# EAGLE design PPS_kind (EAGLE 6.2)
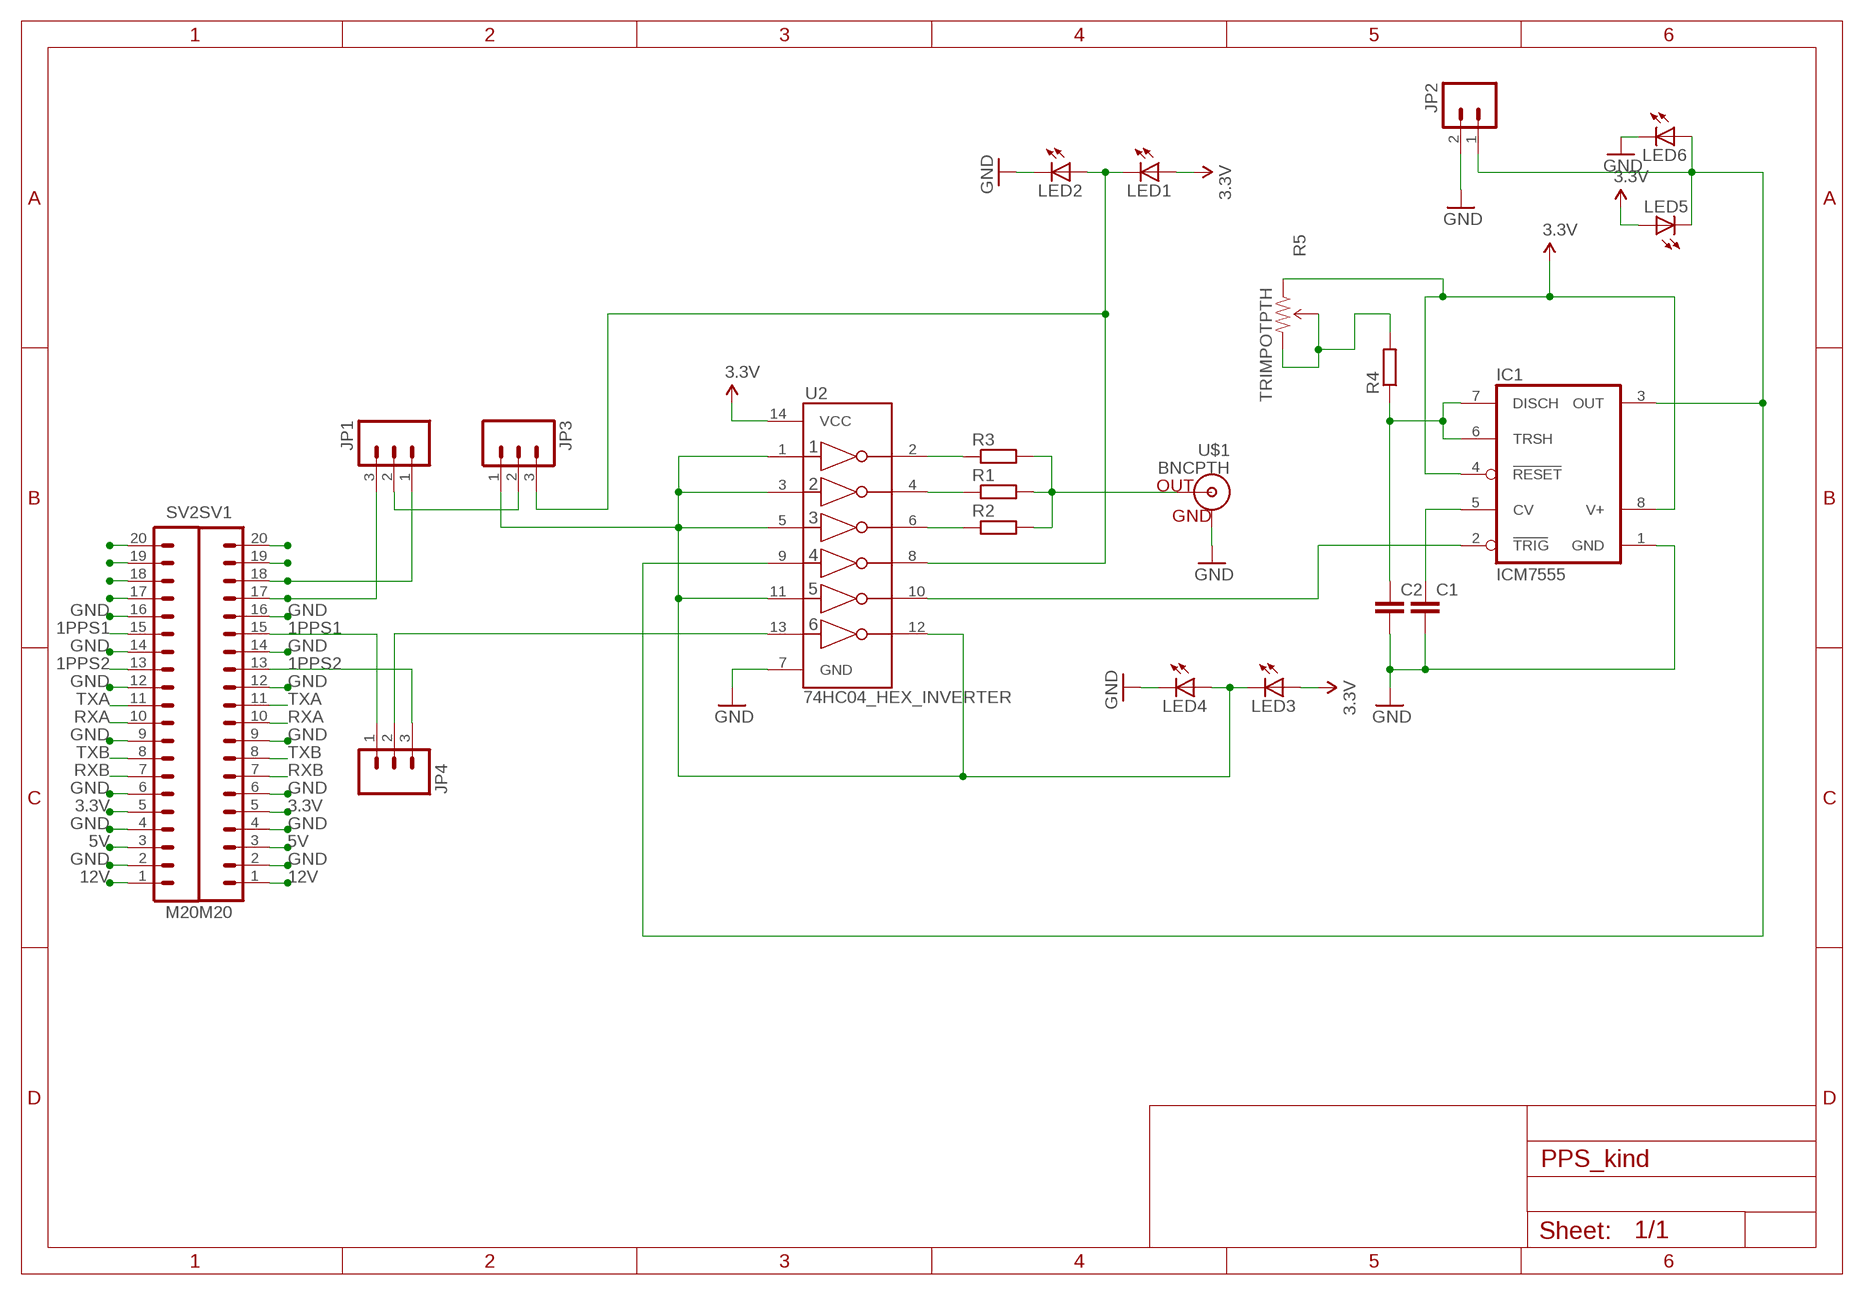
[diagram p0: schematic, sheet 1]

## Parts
C1  CAPPTH1  [CAP-PTH-5MM]
C2  CAPPTH1  [CAP-PTH-5MM]
IC1  ICM7555  [DIL08]
JP1  M03LONGPADS  [1X03_LONGPADS]
JP2  M02PTH3  [1X02_LONGPADS]
JP3  M03LONGPADS  [1X03_LONGPADS]
JP4  M03LONGPADS  [1X03_LONGPADS]
LED1  LED5MM  [LED5MM]
LED2  LED5MM  [LED5MM]
LED3  LED5MM  [LED5MM]
LED4  LED5MM  [LED5MM]
LED5  LED5MM  [LED5MM]
LED6  LED5MM  [LED5MM]
R1  R-EU_0207/10  [0207/10]
R2  R-EU_0207/10  [0207/10]
R3  R-EU_0207/10  [0207/10]
R4  R-EU_0204/2V  [0204V]
R5  TRIMPOTPTH  [TRIM_POT_PTH]
SV1  M20  [1X20]
SV2  M20  [1X20]
U2  74HC04_HEX_INVERTER  [DIL14]
U$1  BNCPTH  [BNC]

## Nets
1PPS1: JP4.1 SV1.15 SV2.15
1PPS2: JP4.3 SV1.13 SV2.13
3.3V: IC1.4(RESET) IC1.8(V+) LED1.A LED3.A LED5.A R5.1(CCW) SV1.5 SV2.5 U2.14(VCC)
5V: SV1.3 SV2.3
12V: SV1.1 SV2.1
GND: C1.2 C2.2 IC1.1(GND) JP2.2 LED2.K(C) LED4.K(C) LED6.K(C) SV1.2 SV1.4 SV1.6 SV1.9 SV1.12 SV1.14 SV1.16 SV2.2 SV2.4 SV2.6 SV2.9 SV2.12 SV2.14 SV2.16 U2.7(GND) U$1.GND
N$1: C1.1 IC1.5(CV)
N$2: JP4.2 U2.13(6A)
N$3: SV2.17
N$4: SV2.18
N$5: SV2.19
N$6: SV2.20
N$8: IC1.2(TRIG) U2.10(5Y)
N$9: JP3.1 LED3.K(C) LED4.A U2.1(1A) U2.3(2A) U2.5(3A) U2.11(5A) U2.12(6Y)
N$10: JP1.2 JP3.2
N$11: IC1.3(OUT) JP2.1 LED5.K(C) LED6.A U2.9(4A)
N$12: JP3.3 LED1.K(C) LED2.A U2.8(4Y)
N$13: R4.2 R5.2(WIPER) R5.3(CW)
N$15: R1.1 U2.4(2Y)
N$16: R2.1 U2.6(3Y)
N$17: JP1.3 SV1.17
N$18: JP1.1 SV1.18
N$19: SV1.19
N$20: SV1.20
N$21: R3.1 U2.2(1Y)
N$24: R1.2 R2.2 R3.2 U$1.S(OUT)
N$25: C2.1 IC1.6(TRSH) IC1.7(DISCH) R4.1
RXA: SV1.10 SV2.10
RXB: SV1.7 SV2.7
TXA: SV1.11 SV2.11
TXB: SV1.8 SV2.8

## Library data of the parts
C1 C2 = SparkFun:CAP: Capacitor
IC1 = maxim:ICM7555: TIMER; MF: MAXIM; MPN: ICM7555IPA+; OC_FARNELL: 9663762; OC_NEWARK: 68K4387
JP1 JP3 JP4 = SparkFun:M03: Header 3 Standard 3-pin 0.1" header. Use with straight break away headers (SKU : PRT-00116), right angle break away headers (PRT-00553), swiss pins (PRT-00743), machine pins (PRT-00117), and female headers (PRT-00115). Molex polarized connector foot print use with SKU : PRT-08232 with associated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
JP2 = SparkFun:M02: Header 2
LED1-LED6 = SparkFun:LED: LEDs
R1-R4 = rcl:R-EU_: RESISTOR, European symbol
R5 = SparkFun:TRIMPOT
SV1 SV2 = SparkFun:M20: This is just like the LOCK variant in that the holes are staggared by 5 mil, but except for the last two holes. They are not altered from the "standard" footprint layout. This is used for a special purpose on the layout of our Graphic LCD Backpack. Make sure you want to use this device before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
U2 = SparkFun:74HC04_HEX_INVERTER: 74HC04 Hex Inverter
U$1 = SparkFun:BNC: BNC Connector, Mouser Part# 5227161

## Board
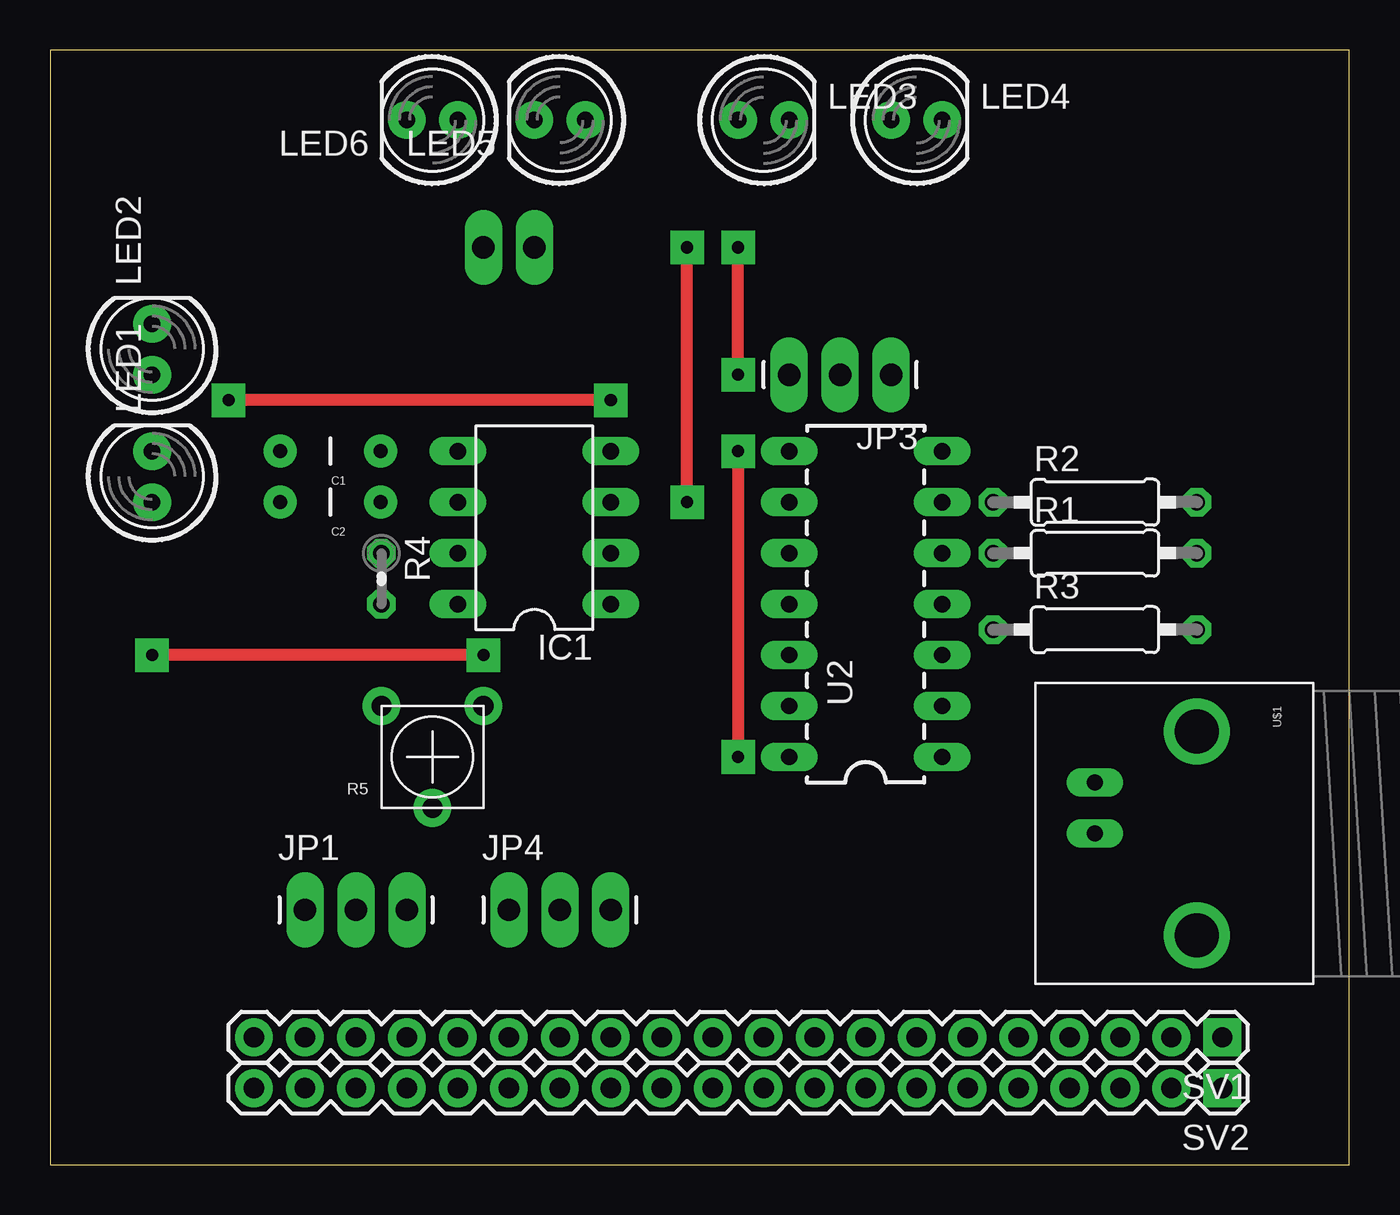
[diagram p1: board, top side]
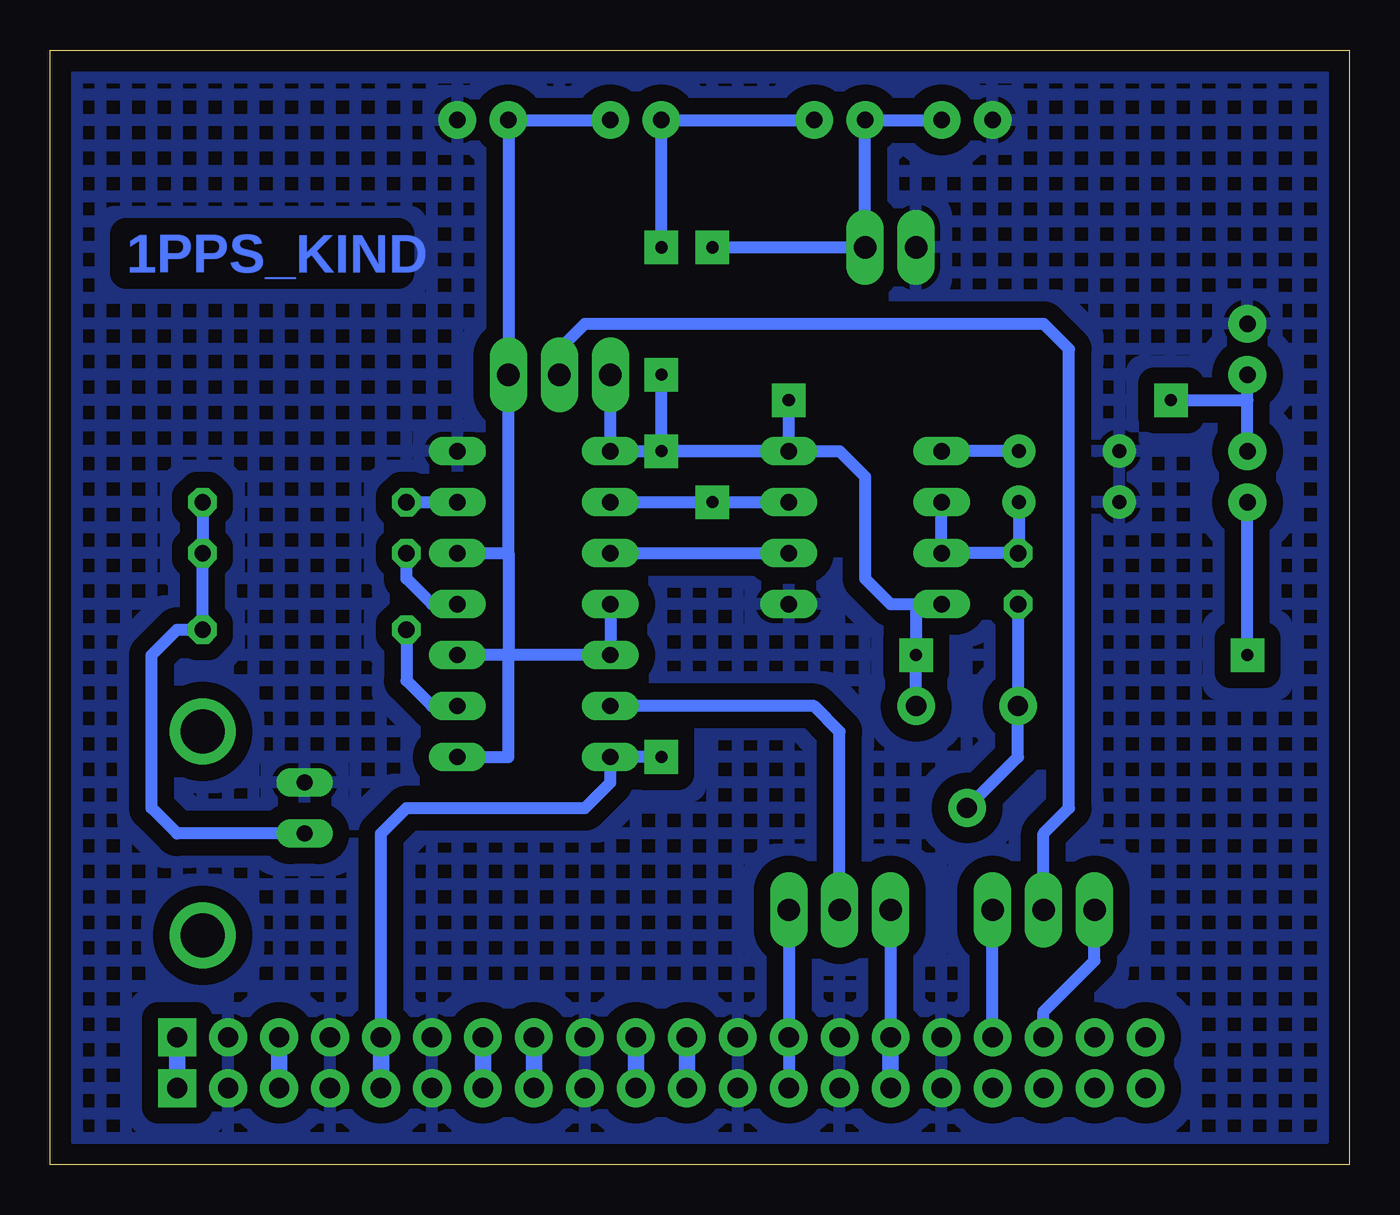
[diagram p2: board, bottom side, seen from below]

Size 64.75 x 55.55 mm. Coordinates in mm from the lower left corner, seen from the top.
Outline: 0,0 64.75,0 64.75,55.55 0,55.55 0,0
Copper layers (1*16): Top 0.035mm / dielectric 1.5mm / Bottom 0.035mm
Design rules: minimum track width 10mil, minimum drill 24mil, track to track 8mil, track to pad 8mil, pad to pad 8mil, via to via 8mil, smd to smd 8mil, copper to edge 40mil, drill to drill 8mil, minimum pad ring 12mil, minimum via ring 12mil, stop-mask expansion 4mil, vias tented up to drill 0mil, thermal gap 10mil

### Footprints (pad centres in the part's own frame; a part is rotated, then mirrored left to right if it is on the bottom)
CAP-PTH-5MM = drill 0.7 pad 1.651: 1 -2.5,0; 2 2.5,0
DIL08 = drill 0.813 long: 1 -3.81,-3.81; 2 -1.27,-3.81; 3 1.27,-3.81; 4 3.81,-3.81; 5 3.81,3.81; 6 1.27,3.81; 7 -1.27,3.81; 8 -3.81,3.81
1X03_LONGPADS = drill 1.118 pad 1.88 long: 1 0,0; 2 2.54,0; 3 5.08,0
1X02_LONGPADS = drill 1.118 pad 1.88 long: 1 0,0; 2 2.54,0
LED5MM = drill 0.813 pad 1.88: A -1.27,0; K 1.27,0
0207/10 = drill 0.813 octagon: 1 -5.08,0; 2 5.08,0
0204V = drill 0.813 octagon: 1 -1.27,0; 2 1.27,0
TRIM_POT_PTH = drill 1 pad 1.88: 1 -2.54,-2.54; 2 0,2.54; 3 2.54,-2.54
1X20 = drill 1.016 pad 1.88 square: 1 0,0 | drill 1.016 pad 1.88: 2 2.54,0; 3 5.08,0; 4 7.62,0; 5 10.16,0; 6 12.7,0; 7 15.24,0; 8 17.78,0; 9 20.32,0; 10 22.86,0; 11 25.4,0; 12 27.94,0; 13 30.48,0; 14 33.02,0; 15 35.56,0; 16 38.1,0; 17 40.64,0; 18 43.18,0; 19 45.72,0; 20 48.26,0
DIL14 = drill 0.813 long: 1 -8.89,-3.81; 2 -6.35,-3.81; 3 -3.81,-3.81; 4 -1.27,-3.81; 5 1.27,-3.81; 6 3.81,-3.81; 7 6.35,-3.81; 8 6.35,3.81; 9 3.81,3.81; 10 1.27,3.81; 11 -1.27,3.81; 12 -3.81,3.81; 13 -6.35,3.81; 14 -8.89,3.81
BNC = drill 2.2: 3 -5.08,5.08; 4 5.08,5.08 | drill 0.8 long: GND -2.54,0; S 0,0

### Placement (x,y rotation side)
C1  13.97,35.56 180 top
C2  13.97,33.02 180 top
IC1  24.13,31.75 90 top
JP1  12.7,12.7 0 top
JP2  24.13,45.72 180 top
JP3  41.91,39.37 180 top
JP4  22.86,12.7 0 top
LED1  5.08,34.29 90 top
LED2  5.08,40.64 90 top
LED3  35.56,52.07 0 top
LED4  43.18,52.07 0 top
LED5  25.4,52.07 180 top
LED6  19.05,52.07 180 top
R1  52.07,30.48 0 top
R2  52.07,33.02 0 top
R3  52.07,26.67 0 top
R4  16.51,29.21 270 top
R5  19.05,20.32 180 top
SV1  58.42,6.35 180 top
SV2  58.42,3.81 180 top
U2  40.64,29.21 90 top
U$1  52.07,16.51 270 top

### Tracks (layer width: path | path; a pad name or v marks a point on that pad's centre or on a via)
1PPS1
  Bottom 0.61: JP4.1 SV2.15
  Bottom 0.813: SV1.15 SV2.15
1PPS2
  Bottom 0.61: JP4.3 SV1.13 SV2.13
3.3V  (via drill 0.6, 0.6 pad 1.68)
  Top 0.61: v34.29,35.56 v34.29,20.32 | v21.59,25.4 v5.08,25.4 | v34.29,39.37 v34.29,45.72
  Bottom 0.61: v34.29,20.32 U2.14 36.83,19.05 38.1,17.78 46.99,17.78 48.26,16.51 SV1.5 | 21.59,27.94 22.86,27.94 24.13,29.21 24.13,34.29 25.4,35.56 IC1.4 v34.29,35.56 v34.29,39.37 | R5.1 v21.59,25.4 21.59,27.94 | LED5.A LED3.A v34.29,45.72 | IC1.8 21.59,27.94 | v5.08,25.4 LED1.A
  Bottom 0.813: SV1.5 SV2.5
5V
  Bottom 0.813: SV1.3 SV2.3
12V
  Bottom 0.813: SV1.1 SV2.1
GND
  pour Bottom (isolate 0.813, hatched): 1.27,1.27 1.27,54.61 63.5,54.61 63.5,1.27
N$1
  Bottom 0.61: C1.1 IC1.5
N$2
  Bottom 0.61: JP4.2 25.4,21.59 26.67,22.86 U2.13
N$8
  Bottom 0.61: U2.10 IC1.2
N$9
  Bottom 0.61: 41.91,25.4 U2.12 U2.11 | 41.91,25.4 U2.3 | U2.5 41.91,30.48 | 41.91,30.48 41.91,25.4 | U2.1 41.91,20.32 41.91,25.4 | 41.91,30.48 JP3.1 LED4.A LED3.K
N$10
  Bottom 0.61: JP1.2 15.24,16.51 13.97,17.78 13.97,40.64 15.24,41.91 38.1,41.91 39.37,40.64 JP3.2
N$11  (via drill 0.6, 0.6 pad 1.68)
  Top 0.61: v31.75,33.02 v31.75,45.72
  Bottom 0.61: U2.9 v31.75,33.02 IC1.3 | LED6.A LED5.K JP2.1 v31.75,45.72
N$12  (via drill 0.6, 0.6 pad 1.68)
  Top 0.61: v27.94,38.1 v8.89,38.1
  Bottom 0.61: JP3.3 U2.8 27.94,35.56 v27.94,38.1 | v8.89,38.1 5.08,38.1 | 5.08,38.1 LED2.A | LED1.K 5.08,38.1
N$13
  Bottom 0.61: R4.2 R5.3 16.51,20.32 R5.2
N$15
  Bottom 0.61: U2.4 45.72,27.94 46.99,29.21 R1.1
N$16
  Bottom 0.61: R2.1 U2.6
N$17
  Bottom 0.61: SV1.17 JP1.3
N$18
  Bottom 0.61: SV1.18 15.24,7.62 12.7,10.16 JP1.1
N$21
  Bottom 0.61: R3.1 46.99,24.13 45.72,22.86 U2.2
N$24
  Bottom 0.61: R2.2 R1.2 R3.2 58.42,26.67 59.69,25.4 59.69,17.78 58.42,16.51 U$1.S
N$25
  Bottom 0.61: C2.1 16.47,30.48 R4.1 IC1.7 IC1.6
RXA
  Bottom 0.813: SV1.10 SV2.10
RXB
  Bottom 0.813: SV1.7 SV2.7
TXA
  Bottom 0.813: SV1.11 SV2.11
TXB
  Bottom 0.813: SV1.8 SV2.8

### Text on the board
Bottom: 1PPS_KIND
